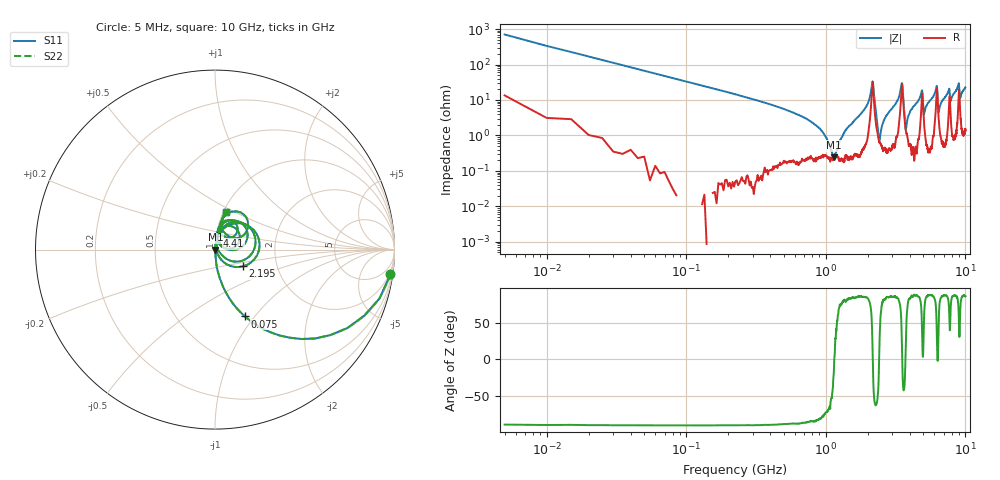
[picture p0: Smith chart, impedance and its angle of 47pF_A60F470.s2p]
! Amotech Co.,Ltd.
! http://www.amotech.co.kr/
! Part Number: A60F470
! These Parameters are Measured in Series Mode Connection
! Operation Temp=25[degC], DC Bias Voltage=0[V]
! Freq. Start=5[MHz] Stop=10[GHz], 2000[Steps]
! Date: Monday, July 20, 2020, 04:22:09
# GHZ S RI R 50.000000
!Freq.(Hz) S11(Real) S11(Imag) S21(Real) S21(Imag) S12(Real) S12(Imag) S22(Real) S22(Imag)
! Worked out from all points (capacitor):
!   2000 points, 5 MHz to 10 GHz, reference 50 ohm
!   read as one part in series: C = 47.2 pF near 55 MHz
!   lowest |Z| = 239 mohm at 1.145 GHz (marker M1)
!   series resonance near 1.15 GHz, so ESL is about 410 pH
!   S11 on the Smith chart (normalised r, x): 5 MHz: 1, -14; 75 MHz: 1.00, -0.90; 2.195 GHz: 1.34, -0.26; 4.41 GHz: 1.01, +0.16; 10 GHz: 1.03, +0.45
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0.005  0.9776 -0.1387  0.0224 0.1387  0.0224 0.1387  0.9776 -0.1387
0.075  0.1672 -0.3726  0.8328 0.3726  0.8328 0.3726  0.1672 -0.3726
0.28  0.0133 -0.1121  0.9867 0.1121  0.9867 0.1121  0.0133 -0.1121
0.905  0.00261 -0.0154  0.9974 0.0154  0.9974 0.0154  0.00261 -0.0154
1.145  0.00234 -0.000479  0.9977 0.000479  0.9977 0.000479  0.00234 -0.000479
1.675  0.00381 0.0312  0.9962 -0.0312  0.9962 -0.0312  0.00381 0.0312
2.195  0.1564 -0.0934  0.8436 0.0934  0.8436 0.0934  0.1564 -0.0934
2.425  0.00648 0.00277  0.9935 -0.00277  0.9935 -0.00277  0.00648 0.00277
2.67  0.00533 0.0315  0.9947 -0.0315  0.9947 -0.0315  0.00533 0.0315
3.34  0.033 0.1123  0.967 -0.1123  0.967 -0.1123  0.033 0.1123
3.52  0.2241 0.0219  0.7759 -0.0219  0.7759 -0.0219  0.2241 0.0219
3.745  0.0135 0.00638  0.9865 -0.00638  0.9865 -0.00638  0.0135 0.00638
4.41  0.0105 0.0768  0.9895 -0.0768  0.9895 -0.0768  0.0105 0.0768
4.87  0.1132 0.1192  0.8868 -0.1192  0.8868 -0.1192  0.1132 0.1192
5.005  0.04 0.0156  0.96 -0.0156  0.96 -0.0156  0.04 0.0156
6.205  0.1467 0.1479  0.8533 -0.1479  0.8533 -0.1479  0.1467 0.1479
6.415  0.0352 0.0256  0.9648 -0.0256  0.9648 -0.0256  0.0352 0.0256
6.67  0.0148 0.0773  0.9852 -0.0773  0.9852 -0.0773  0.0148 0.0773
8.335  0.0323 0.1515  0.9677 -0.1515  0.9677 -0.1515  0.0323 0.1515
8.945  0.1561 0.1985  0.8439 -0.1985  0.8439 -0.1985  0.1561 0.1985
9.17  0.0574 0.089  0.9426 -0.089  0.9426 -0.089  0.0574 0.089
10  0.061 0.208  0.939 -0.208  0.939 -0.208  0.061 0.208
